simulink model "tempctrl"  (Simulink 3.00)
settings: Solver=ode45  StartTime=0.0  StopTime=500  RelTol=1e-3

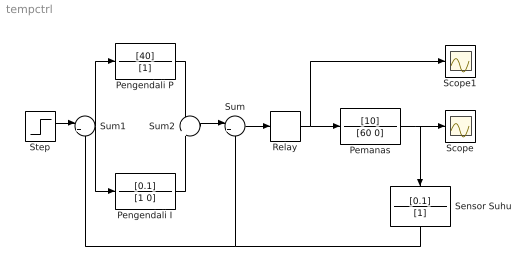
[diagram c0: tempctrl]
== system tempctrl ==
  Pemanas : TransferFcn  Numerator=[10]  Denominator=[60 0]
  Pengendali I : TransferFcn  Numerator=[0.1]  Denominator=[1 0]
  Pengendali P : TransferFcn  Numerator=[40]  Denominator=[1]
  Relay : Relay  OnSwitchValue=1  OffSwitchValue=-1  OnOutputValue=1  OffOutputValue=-1
  Scope : Scope
  Scope1 : Scope
  Sensor Suhu : TransferFcn  Orientation=down  Numerator=[0.1]  Denominator=[1]
  Step : Step  Time=1  Before=0  After=1  SampleTime=0
  Sum : Sum  Inputs=|+-  SaturateOnIntegerOverflow=on
  Sum1 : Sum  Inputs=|+-  SaturateOnIntegerOverflow=on
  Sum2 : Sum  Inputs=+||+  SaturateOnIntegerOverflow=on
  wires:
  Sum/1 -> Relay/1
  Step/1 -> Sum1/1
  Relay/1 -> Pemanas/1, Scope1/1
  Sum1/1 -> Pengendali I/1, Pengendali P/1
  Sum2/1 -> Sum/1
  Pengendali I/1 -> Sum2/2
  Pengendali P/1 -> Sum2/1
  Sensor Suhu/1 -> Sum1/2, Sum/2
  Pemanas/1 -> Scope/1, Sensor Suhu/1
